(* Action node that extends base node *)
FUNCTION_BLOCK FB_ActionNode EXTENDS FB_BaseNode
VAR
    _nExecutionCount : INT;
    _bFirstExecution : BOOL := TRUE;
END_VAR

METHOD Tick : E_NodeStatus
IF _bFirstExecution THEN
    _bFirstExecution := FALSE;
    _nExecutionCount := 0;
END_IF

_nExecutionCount := _nExecutionCount + 1;

IF HasError() THEN
    Tick := E_NodeStatus.FAILURE;
ELSE
    Tick := E_NodeStatus.SUCCESS;
END_IF

eLastStatus := Tick;
END_METHOD

METHOD Reset : BOOL
SUPER^.Reset();
_nExecutionCount := 0;
_bFirstExecution := TRUE;
Reset := TRUE;
END_METHOD

METHOD PUBLIC GetExecutionCount : INT
GetExecutionCount := _nExecutionCount;
END_METHOD

END_FUNCTION_BLOCK
